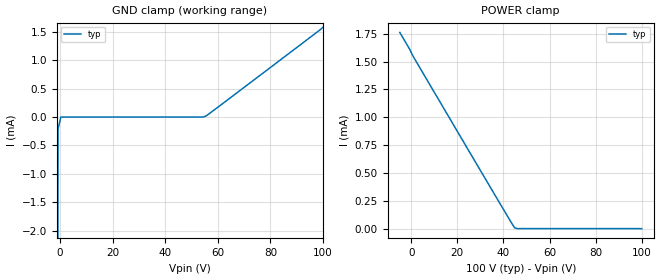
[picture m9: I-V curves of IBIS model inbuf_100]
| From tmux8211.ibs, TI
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| inbuf_100
[Model]   inbuf_100
Model_type   Input
Vinl = 0.8
Vinh = 1.3
|   typ   min   max
C_comp   1.598234e-13   NA   NA
[Voltage Range]   100   NA   NA
[Temperature Range]   27   NA   NA
[Power Clamp Reference]   100   NA   NA
[GND Clamp Reference]   0   NA   NA
[GND Clamp]
|   Voltage   I(typ)   I(min)   I(max)
-5V       -116.5mA   NA         NA
-1.818V   -26.13mA   NA         NA
-757.6mV  -207.5uA   NA         NA
303mV     62.34nA    NA         NA
54.39V    555.2nA    NA         NA
55.45V    16.93uA    NA         NA
100V      1.582mA    NA         NA
[POWER Clamp]
|   Voltage   I(typ)   I(min)   I(max)
-5V       1.762mA    NA         NA
-758mV    1.613mA    NA         NA
1.364V    1.527mA    NA         NA
44.85V    7.413uA    NA         NA
45.91V    555.2nA    NA         NA
100V      -220pA     NA         NA
